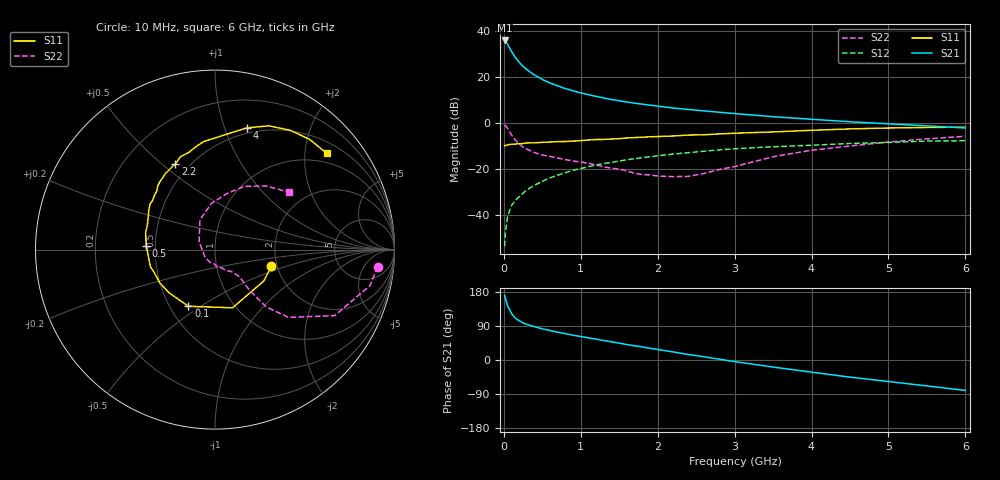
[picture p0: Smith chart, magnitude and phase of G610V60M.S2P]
! SIEMENS Small Signal Semiconductors
! BFG193
! Si NPN RF Bipolar Junction Transistor in SOT223
! VCE = 10 V  IC = 60 mA
! Common Emitter S-Parameters:  August  1996
# GHz  S  MA  R  50
!  f  S11  S21  S12  S22
! GHz  MAG  ANG  MAG  ANG  MAG  ANG  MAG  ANG
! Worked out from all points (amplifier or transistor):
!   36 points, 10 MHz to 6 GHz, reference 50 ohm
!   highest |S21| = 36.1 dB at 10 MHz (marker M1)
!   |S21| within 3 dB of that: start of sweep to 70.23 MHz
!   unconditionally stable (mu >= 1): 452.8 MHz to 2.392 GHz
!   at 250 MHz: K = 0.91, MSG = 27.6 dB, |S12| = -30.4 dB
!   at 1.4 GHz: K = 1.04, MAG = 12.4 dB, |S12| = -17.0 dB
!   at 6 GHz: K = 0.89, MSG = 2.8 dB, |S12| = -7.6 dB
!   S11 on the Smith chart (normalised r, x): 10 MHz: 1.86, -0.39; 100 MHz: 0.62, -0.45; 500 MHz: 0.45, +0.02; 2.2 GHz: 0.42, +0.56; 4 GHz: 0.45, +1.19; 6 GHz: 0.75, +2.49
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0.01  0.3274 -16.7  63.48 170.5  0.0021 81.5  0.9104 -6.0
0.02  0.3235 -32.8  61.08 163.1  0.0041 74.9  0.8874 -13.0
0.05  0.3387 -73.3  51.67 142.4  0.0097 69.6  0.7612 -28.9
0.1  0.3486 -115.1  36.59 122.6  0.0162 65.3  0.5571 -42.7
0.15  0.3518 -137.1  26.92 110.3  0.0208 65.0  0.4279 -48.2
0.2  0.3593 -149.3  21.22 103.4  0.0251 67.0  0.355 -49.0
0.25  0.3611 -158.6  17.34 98.0  0.0301 66.9  0.3022 -49.4
0.3  0.3721 -165.0  14.67 94.0  0.0355 68.5  0.2724 -49.5
0.4  0.3735 -174.9  11.17 88.0  0.0447 68.9  0.2285 -48.5
0.5  0.3834 177.1  8.964 82.2  0.0542 68.0  0.2033 -48.1
0.6  0.3895 171.1  7.538 77.8  0.0644 67.2  0.1885 -48.9
0.8  0.3997 161.1  5.676 69.4  0.084 64.3  0.1611 -52.2
1.1  0.4308 148.7  4.173 58.4  0.1133 59.2  0.1337 -61.8
1.3  0.4426 141.9  3.544 51.4  0.1322 55.2  0.1121 -68.4
1.6  0.4774 131.9  2.891 40.8  0.1598 48.4  0.0916 -86.4
2.2  0.5271 114.7  2.146 21.2  0.2126 35.1  0.0686 -143.9
2.8  0.5851 100.1  1.734 2.2  0.2627 21.3  0.0983 153.9
3.5  0.6462 84.2  1.388 -18.6  0.3074 4.2  0.1864 116.7
4  0.7013 75.3  1.219 -32.1  0.3315 -5.6  0.2578 94.5
4.5  0.752 66.5  1.076 -45.2  0.3623 -15.8  0.3195 77.9
5.5  0.8093 49.3  0.875 -68.4  0.4086 -39.0  0.4564 50.9
6  0.8218 40.8  0.788 -80.3  0.4153 -52.4  0.52 38.0
